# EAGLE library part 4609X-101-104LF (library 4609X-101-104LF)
Resistor Networks & Arrays 9pins 100Kohms Bussed Source: Datasheet
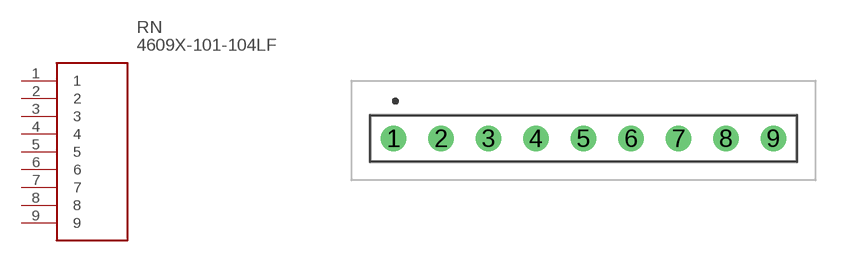
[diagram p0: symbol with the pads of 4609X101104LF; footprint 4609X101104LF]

Designator prefix RN

## 4609X-101-104LF (Description: Resistor Networks & Arrays 9pins 100Kohms Bussed; Height: 5.08mm; Manufacturer_Name: Bourns; Manufacturer_Part_Number: 4609X-101-104LF)  [4609X101104LF]
1  1
2  2
3  3
4  4
5  5
6  6
7  7
8  8
9  9

## Footprint 4609X101104LF (pad centres in mm)
4609X-101-104LF-1
drill 0.84 pad 1.365: 1 0,0; 2 2.54,0; 3 5.08,0; 4 7.62,0; 5 10.16,0; 6 12.7,0; 7 15.24,0; 8 17.78,0; 9 20.32,0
